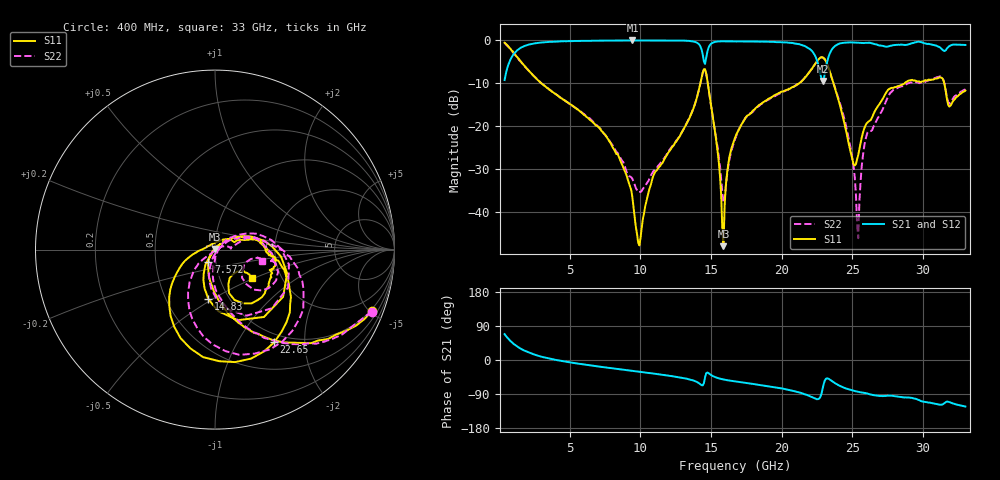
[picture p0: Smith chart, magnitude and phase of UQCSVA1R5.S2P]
!  Part Number  UQCSVA1R5  Mounting Orientation: Horizontal
!  Description: Ultra Low ESR Microwave capacitors
!  Application: Coupling, Bypass, Tuning, DC Block
!  Filters, Matching
# GHZ S DB R 50
! Freq  |S11|  S11 Ph  |S21|  S21 Ph  |S12|  S12 Ph  |S22|  S22 Ph
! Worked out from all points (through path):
!   401 points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, 400 MHz to 33 GHz, reference 50 ohm
!   highest |S21| = 0.00 dB at 9.447 GHz (marker M1); lowest = -9.5 dB at 22.89 GHz (marker M2)
!   group delay of S21, straight-line fit = 11.9 ps
!   lowest |S11| = -47.9 dB at 15.88 GHz (marker M3), VSWR 1.01, Z = 50.1 + j0.398 ohm
!   |S11| at or under -10 dB: 3.004 GHz to 14.25 GHz (11.24 GHz wide, 130 % of centre); 14.78 GHz to 21.23 GHz (6.456 GHz wide, 35.9 % of centre); 23.67 GHz to 28.7 GHz (5.026 GHz wide, 19.2 % of centre)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
!   |S22| runs from -46.1 to -0.5 dB; largest |S21 - S12| = 0.014
!   S11 on the Smith chart (normalised r, x): 400 MHz: 0.89, -5.17; 7.572 GHz: 0.92, -0.13; 14.83 GHz: 0.80, -0.48; 22.65 GHz: 0.87, -1.44; 33 GHz: 1.43, -0.48
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0.4  -0.54 -21.3  -9.22 68.2  -9.19 68.1  -0.55 -21.6
2.193  -7.34 -72.1  -0.90 18.5  -0.91 18.0  -7.36 -70.9
5.861  -16.84 -104.4  -0.10 -11.0  -0.09 -11.0  -16.76 -94.8
7.572  -22.19 -118.2  -0.03 -19.8  -0.04 -19.9  -22.32 -93.3
9.447  -36.70 -148.9  0.00 -28.8  -0.02 -28.8  -32.28 -61.7
9.936  -47.72 131.3  -0.01 -31.0  -0.01 -31.0  -35.29 -26.4
11.321  -29.52 48.0  -0.01 -37.7  -0.01 -37.6  -29.00 30.4
14.337  -8.63 -6.1  -2.12 -66.4  -2.11 -66.1  -8.70 0.9
14.826  -11.10 -97.5  -1.70 -34.7  -1.72 -35.2  -11.26 -88.2
15.885  -47.91 80.9  -0.20 -51.5  -0.19 -51.5  -37.80 -44.0
16.7  -22.72 39.2  -0.22 -56.6  -0.19 -56.7  -23.02 32.3
22.161  -6.51 -28.3  -2.52 -97.8  -2.52 -97.8  -6.45 -13.0
22.65  -4.25 -57.5  -6.51 -102.0  -6.47 -101.4  -4.33 -39.1
22.894  -3.92 -79.9  -9.45 -76.5  -9.34 -76.4  -3.94 -61.0
23.465  -7.87 -129.1  -2.63 -53.2  -2.65 -53.3  -7.83 -108.2
24.524  -20.48 -174.6  -0.49 -74.9  -0.53 -74.7  -19.41 -139.8
25.095  -28.94 130.2  -0.46 -81.2  -0.49 -80.9  -29.52 -134.3
25.421  -26.66 71.8  -0.53 -84.1  -0.56 -83.5  -46.06 -17.0
25.991  -19.39 28.5  -0.56 -87.8  -0.58 -87.7  -22.33 12.2
27.621  -11.31 4.8  -1.30 -94.2  -1.35 -94.0  -12.54 14.9
31.452  -9.36 -61.8  -2.36 -115.5  -2.38 -115.7  -9.22 -41.2
33  -11.67 -37.3  -1.05 -122.8  -1.08 -122.5  -11.43 -13.6
